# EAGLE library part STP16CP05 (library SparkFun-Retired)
16-pin constant current sink shift register LED driver Not in catalog
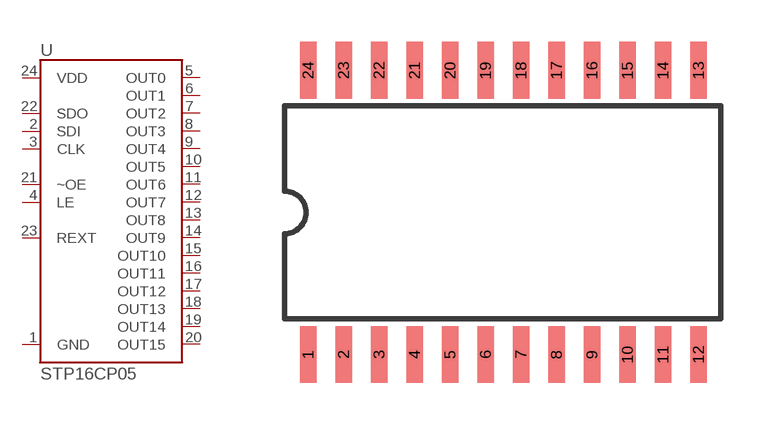
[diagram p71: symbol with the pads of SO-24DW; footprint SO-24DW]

Designator prefix -

## STP16CP05  [SO-24DW]
1  GND
2  SDI
3  CLK
4  LE
5  OUT0
6  OUT1
7  OUT2
8  OUT3
9  OUT4
10  OUT5
11  OUT6
12  OUT7
13  OUT8
14  OUT9
15  OUT10
16  OUT11
17  OUT12
18  OUT13
19  OUT14
20  OUT15
21  ~OE
22  SDO
23  REXT
24  VDD

## Footprint SO-24DW (pad centres in mm)
300-mil body, package type SO
smd 0.584 x 2.032: 1 -6.35,-5.08; 2 -5.08,-5.08; 3 -3.81,-5.08; 4 -2.54,-5.08; 5 -1.27,-5.08; 6 0,-5.08; 7 1.27,-5.08; 8 2.54,-5.08; 9 3.81,-5.08; 10 5.08,-5.08; 11 6.35,-5.08; 12 7.62,-5.08; 13 7.62,5.08; 14 6.35,5.08; 15 5.08,5.08; 16 3.81,5.08; 17 2.54,5.08; 18 1.27,5.08; 19 0,5.08; 20 -1.27,5.08; 21 -2.54,5.08; 22 -3.81,5.08; 23 -5.08,5.08; 24 -6.35,5.08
